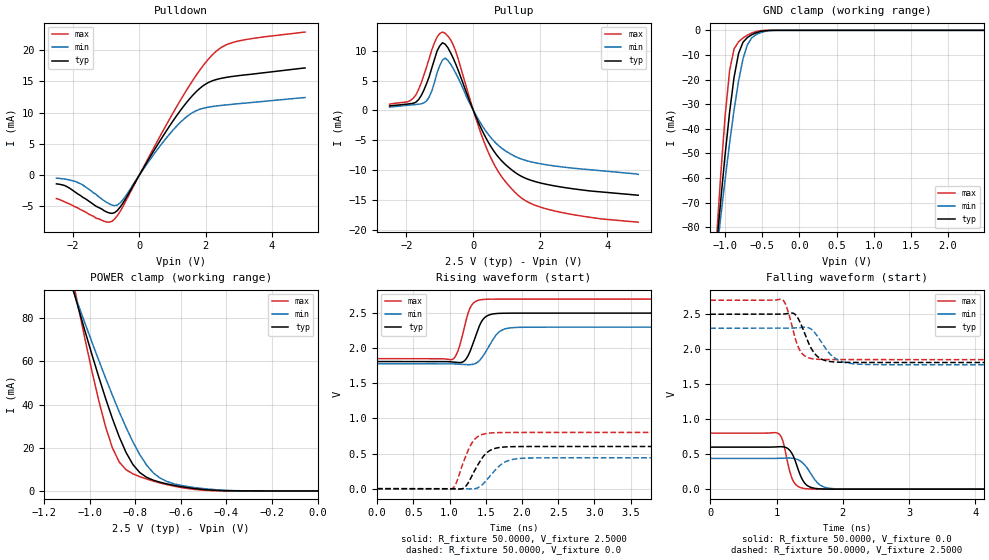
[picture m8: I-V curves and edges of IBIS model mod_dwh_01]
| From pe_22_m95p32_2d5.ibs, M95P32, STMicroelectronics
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|   Model mod_dwh_01
[Model]   mod_dwh_01
Model_type I/O
Polarity   Non-Inverting
Enable   Active-High
Vinl   =   0.750V
Vinh   =   1.750V
Vmeas  =   1.250V
Cref   =   30.0pF
C_comp   1.219pF   1.164pF   1.337pF
[Model Spec]
Vinl   0.750V  0.690V  0.810V  | <- for Vcc = 2.5V, 2.3V, 2.7V
Vinh   1.750V  1.610V  1.890V  | <- for Vcc = 2.5V, 2.3V, 2.7V
Vmeas  1.250V  1.150V  1.350V  | <- for Vcc = 2.5V, 2.3V, 2.7V
[Temperature Range]  25.0000   0.1050k   -40.0000
[Voltage Range]   2.5000V   2.3000V   2.7000V
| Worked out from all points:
|   slope of the pulldown table from 0 to 0.375 V, typ, clamps not added: 112 ohm
|   slope of the pullup table from 0 to 0.375 V, typ, clamps not added: 81.3 ohm
|   GND clamp passes 1 mA (typ) near -0.58 V on its own axis
|   POWER clamp passes 1 mA (typ) near -0.53 V on its own axis
|   rising waveform, R_fixture 50.0000, V_fixture 2.5000: 20-80 % time 152ps typ, 190ps min, 131ps max; typ from 1.81 V to 2.5 V
|   rising waveform, R_fixture 50.0000, V_fixture 0.0: 20-80 % time 205ps typ, 241ps min, 182ps max; typ from 0 V to 0.601 V
|   falling waveform, R_fixture 50.0000, V_fixture 0.0: 20-80 % time 151ps typ, 202ps min, 123ps max; typ from 0.601 V to 0 V
|   falling waveform, R_fixture 50.0000, V_fixture 2.5000: 20-80 % time 200ps typ, 258ps min, 156ps max; typ from 2.5 V to 1.81 V
[Pulldown]
|Voltage   I(typ)   I(min)   I(max)
-2.5V     -1.4mA     -494uA     -3.75mA
-1.78V    -3.25mA    -1.38mA    -5.5mA
-1.06V    -5.7mA     -4.1mA     -7.39mA
-820mV    -6.119mA   -4.801mA   -7.37mA
-660mV    -5.635mA   -4.778mA   -6.457mA
-500mV    -4.528mA   -3.972mA   -5.081mA
540mV     4.766mA    4.053mA    5.383mA
1.26V     10.48mA    8.543mA    12.14mA
1.74V     13.46mA    10.35mA    16.14mA
2.22V     15.11mA    10.98mA    19.31mA
2.94V     15.86mA    11.4mA     21.37mA
5V        17.13mA    12.4mA     22.86mA
[Pullup]
|Voltage   I(typ)   I(min)   I(max)
-2.5V     762uA      562uA      1.052mA
-1.8V     1.189mA    942uA      2.021mA
-1.4V     4.433mA    1.565mA    7.223mA
-1.08V    10mA       6.346mA    12.32mA
-840mV    11.1mA     8.76mA     12.93mA
-520mV    7.699mA    6.186mA    9.823mA
40mV      -549.1uA   -417.2uA   -720uA
440mV     -5.274mA   -3.974mA   -6.934mA
760mV     -7.918mA   -5.938mA   -10.41mA
1.24V     -10.37mA   -7.693mA   -13.71mA
2.36V     -12.59mA   -9.264mA   -16.77mA
4.92V     -14.22mA   -10.72mA   -18.74mA
[GND_clamp]
|Voltage   I(typ)   I(min)   I(max)
-2.5V     -618.8mA   -507.1mA   -839.7mA
-1.12V    -89.51mA   -92.19mA   -86.51mA
-1.06V    -69.34mA   -76.02mA   -58.94mA
-1V       -50.38mA   -60.48mA   -34.64mA
-940mV    -33.28mA   -45.81mA   -16.38mA
-880mV    -19.11mA   -32.38mA   -7.564mA
-820mV    -9.453mA   -20.71mA   -4.67mA
-760mV    -4.854mA   -11.6mA    -3.093mA
-700mV    -2.891mA   -5.814mA   -1.933mA
-580mV    -964.2uA   -1.685mA   -447.5uA
-340mV    -4.19uA    -39.9uA    -134.6nA
2.48V     343.3pA    931.5nA    131.5pA
[POWER_clamp]
|Voltage   I(typ)   I(min)   I(max)
-2.49V    667.2mA    541mA      921mA
-1.08V    96.07mA    95.11mA    101.2mA
-1.05V    84.91mA    86.28mA    85.45mA
-990mV    63.23mA    68.98mA    55.57mA
-930mV    42.88mA    52.31mA    29.76mA
-900mV    33.53mA    44.31mA    19.96mA
-840mV    17.8mA     29.4mA     9.816mA
-810mV    12.22mA    22.72mA    7.905mA
-750mV    6.305mA    11.96mA    5.516mA
-660mV    3.226mA    4.34mA     2.89mA
-420mV    154.8uA    392.4uA    29.01uA
0V        492.2pA    14.11nA    240.5pA
[Ramp]
| variable   typ   min   max
dV/dt_r   0.3605/0.2740n   0.2726/0.3361n   0.4805/0.2607n
dV/dt_f   0.4139/0.2946n   0.3232/0.3958n   0.5091/0.2611n
R_load = 50.0000
[Rising Waveform]
R_fixture= 50.0000
V_fixture= 2.5000
V_fixture_min= 2.3000
V_fixture_max= 2.7000
|time   V(typ)   V(min)   V(max)
0s        1.81V      1.778V     1.851V
1.04ns    1.804V     1.777V     1.841V
1.12ns    1.796V     1.773V     1.974V
1.2ns     1.816V     1.768V     2.278V
1.28ns    1.948V     1.766V     2.568V
1.344ns   2.128V     1.777V     2.656V
1.456ns   2.403V     1.88V      2.693V
1.664ns   2.495V     2.213V     2.7V
1.888ns   2.5V       2.294V     2.7V
8ns       2.5V       2.3V       2.7V
[Rising Waveform]
R_fixture= 50.0000
V_fixture= 0.0
V_fixture_min= 0.0
V_fixture_max= 0.0
|time   V(typ)   V(min)   V(max)
0s        7.535nV    869nV      1.307nV
1.032ns   -884.5uV   343.5uV    -2.851mV
1.088ns   -3.123mV   173uV      72.95mV
1.2ns     12.91mV    -1.566mV   402.4mV
1.304ns   173.4mV    -4.799mV   643.7mV
1.424ns   397.3mV    33.41mV    760.9mV
1.552ns   540.7mV    174.7mV    791.8mV
1.76ns    593.9mV    376mV      800mV
2.048ns   600.4mV    434.9mV    800.8mV
8ns       600.8mV    439.6mV    800.9mV
[Falling Waveform]
R_fixture= 50.0000
V_fixture= 0.0
V_fixture_min= 0.0
V_fixture_max= 0.0
|time   V(typ)   V(min)   V(max)
0s        600.8mV    439.6mV    800.9mV
1.032ns   606.1mV    440.8mV    792.2mV
1.096ns   605.5mV    442.8mV    687.1mV
1.192ns   562.1mV    444.7mV    282.2mV
1.256ns   467.5mV    439.8mV    110.5mV
1.368ns   180.4mV    396.2mV    21.07mV
1.448ns   64.02mV    320.5mV    6.568mV
1.656ns   4.606mV    60.77mV    336uV
1.896ns   260.9uV    4.943mV    15.88uV
8ns       690.1nV    1.468uV    814.8nV
[Falling Waveform]
R_fixture= 50.0000
V_fixture= 2.5000
V_fixture_min= 2.3000
V_fixture_max= 2.7000
|time   V(typ)   V(min)   V(max)
0s        2.5V       2.3V       2.7V
1.088ns   2.501V     2.3V       2.711V
1.152ns   2.507V     2.3V       2.604V
1.248ns   2.515V     2.302V     2.277V
1.344ns   2.409V     2.308V     2V
1.432ns   2.208V     2.315V     1.901V
1.568ns   1.947V     2.246V     1.86V
1.856ns   1.819V     1.891V     1.852V
2.192ns   1.811V     1.789V     1.851V
8ns       1.81V      1.778V     1.851V
